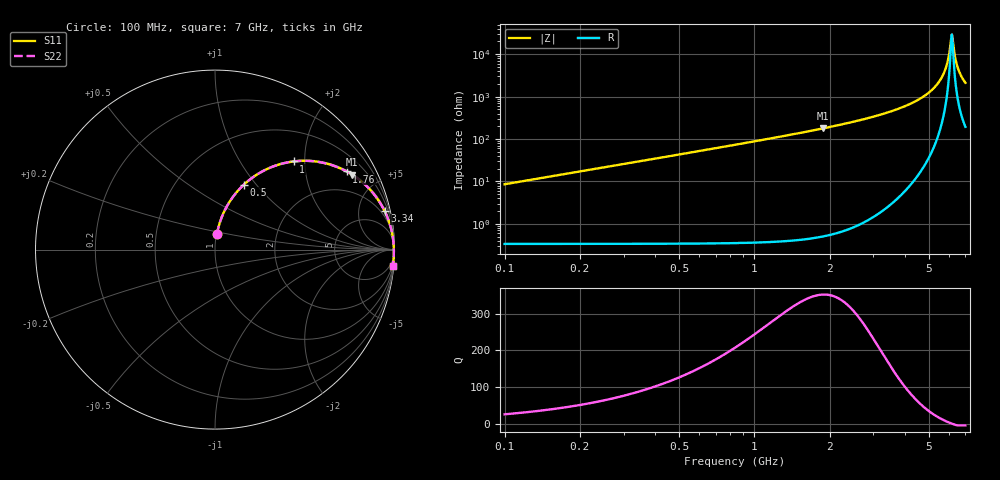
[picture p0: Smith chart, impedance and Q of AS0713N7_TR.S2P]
!AVX Corporation
! PN: AS0713N7*TR
! DESCRIPTION: SQUARE AIR CORE INDUCTOR, 13.7nH, 5 turns
# MHZ S MA R 50
!Freq  MagS11  AngS11  MagS21  AngS21  MagS12  AngS12  MagS22  AngS22
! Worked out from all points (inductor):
!   346 points, 100 MHz to 7 GHz, reference 50 ohm
!   read as one part in series: L = 13.7 nH near 120 MHz
!   highest Q = 353 at 1.88 GHz (marker M1), where L = 15.1 nH
!   self-resonance near 6.16 GHz
!   S11 on the Smith chart (normalised r, x): 100 MHz: 1.01, +0.17; 500 MHz: 1.01, +0.86; 1 GHz: 1.02, +1.77; 1.76 GHz: 1.05, +3.34; 3.34 GHz: 1.24, +8.81; 7 GHz: 1, -22
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100  0.08505 82.8  0.993 -4.9  0.993 -4.9  0.08506 82.8
160  0.1353 80.8  0.9875 -7.8  0.9875 -7.8  0.1353 80.8
260  0.2168 76.5  0.9729 -12.6  0.9729 -12.6  0.2169 76.5
500  0.3944 66.1  0.9158 -23.4  0.9158 -23.4  0.3944 66.1
1000  0.6588 48.2  0.7496 -41.5  0.7496 -41.5  0.6588 48.2
1260  0.7462 41.1  0.6632 -48.7  0.6632 -48.7  0.7462 41.1
1760  0.8527 30.7  0.52 -59.1  0.52 -59.1  0.8527 30.7
1880  0.87 28.7  0.4905 -61.1  0.4905 -61.1  0.8701 28.7
2400  0.9232 21.6  0.3813 -68.2  0.3813 -68.2  0.9233 21.6
3340  0.9695 12.7  0.2396 -77.0  0.2396 -77.0  0.9696 12.7
3560  0.9755 11.1  0.2134 -78.5  0.2134 -78.5  0.9756 11.1
4700  0.9925 4.3  0.1035 -84.5  0.1035 -84.5  0.9925 4.3
5420  0.9961 0.9  0.04926 -86.0  0.04926 -86.0  0.9961 0.9
5680  0.9966 -0.2  0.03166 -84.9  0.03166 -84.9  0.9966 -0.2
5860  0.9967 -0.9  0.02004 -82.0  0.02004 -82.0  0.9967 -0.9
6020  0.9967 -1.6  0.01022 -73.0  0.01022 -73.0  0.9967 -1.6
6140  0.9966 -2.0  0.00408 -36.3  0.00408 -36.3  0.9966 -2.0
6180  0.9966 -2.2  0.003414 0.0  0.003414 0.0  0.9966 -2.2
6340  0.9964 -2.8  0.01033 67.0  0.01033 67.0  0.9964 -2.8
6480  0.9961 -3.3  0.01824 74.9  0.01824 74.9  0.9961 -3.3
6700  0.9956 -4.1  0.03059 78.4  0.03059 78.4  0.9956 -4.1
7000  0.9946 -5.2  0.04689 79.6  0.04689 79.6  0.9946 -5.2
